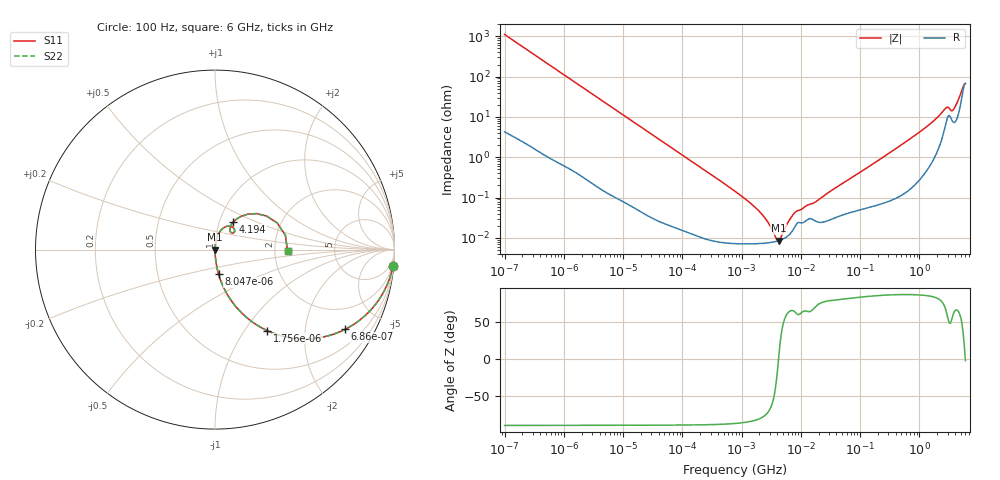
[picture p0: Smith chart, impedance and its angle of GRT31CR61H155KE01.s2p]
!Murata Part Number: GRT31CR61H155KE01
!These Parameters are Measured in Series Mode Connection
!Data Generated on Jun 19, 2026
!  o--ll--o
!Port1  Port2
!  o------o
!Operation Temp=25[degC], DC Bias Voltage=0[V]
!Freq. Start=100[Hz] Stop=6[GHz] 401[Steps]
# Hz S RI R 50
!Freq.(Hz) S11(Real) S11(Imag) S21(Real) S21(Imag) S12(Real) S12(Imag) S22(Real) S22(Imag)
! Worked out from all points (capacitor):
!   401 points, 100 Hz to 6 GHz, reference 50 ohm
!   read as one part in series: C = 1.43 uF near 109 Hz
!   lowest |Z| = 8.57 mohm at 4.246 MHz (marker M1)
!   series resonance near 4.206 MHz, so ESL is about 1 nH
!   S11 on the Smith chart (normalised r, x): 100 Hz: 1, -22; 686 Hz: 1.02, -3.26; 1.756 kHz: 1.01, -1.28; 8.047 kHz: 1.00, -0.28; 4.194 GHz: 1.16, +0.37; 6 GHz: 2.36, -0.05
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100  0.9916 -0.0891  0.00835 0.0891  0.00835 0.0891  0.9916 -0.0891
320  0.9229 -0.2645  0.0771 0.2645  0.0771 0.2645  0.9229 -0.2645
686  0.7258 -0.4436  0.2742 0.4436  0.2742 0.4436  0.7258 -0.4436
1756  0.2912 -0.4514  0.7088 0.4514  0.7088 0.4514  0.2912 -0.4514
2008  0.2395 -0.4238  0.7605 0.4238  0.7605 0.4238  0.2395 -0.4238
3594  0.0907 -0.2842  0.9093 0.2842  0.9093 0.2842  0.0907 -0.2842
8047  0.0202 -0.1373  0.9798 0.1373  0.9798 0.1373  0.0202 -0.1373
40335  0.00105 -0.0281  0.999 0.0281  0.999 0.0281  0.00105 -0.0281
774597  7.41e-05 -0.00143  0.9999 0.00143  0.9999 0.00143  7.41e-05 -0.00143
1983483  7.25e-05 -0.000452  0.9999 0.000452  0.9999 0.000452  7.25e-05 -0.000452
2713602  7.51e-05 -0.000249  0.9999 0.000249  0.9999 0.000249  7.51e-05 -0.000249
3712478  8.11e-05 -6.94e-05  0.9999 6.94e-05  0.9999 6.94e-05  8.11e-05 -6.94e-05
4246196  8.55e-05 5.4e-06  0.9999 -5.4e-06  0.9999 -5.4e-06  8.55e-05 5.4e-06
7947587  0.000191 0.000381  0.9998 -0.000381  0.9998 -0.000381  0.000191 0.000381
1.555665e7  0.000292 0.000647  0.9997 -0.000647  0.9997 -0.000647  0.000292 0.000647
3.124326e8  0.000978 0.0127  0.999 -0.0127  0.999 -0.0127  0.000978 0.0127
1.309207e9  0.00756 0.0556  0.9924 -0.0556  0.9924 -0.0556  0.00756 0.0556
2.679998e9  0.067 0.1299  0.933 -0.1299  0.933 -0.1299  0.067 0.1299
3.666503e9  0.0833 0.1052  0.9167 -0.1052  0.9167 -0.1052  0.0833 0.1052
4.193612e9  0.1023 0.1542  0.8977 -0.1542  0.8977 -0.1542  0.1023 0.1542
5.016141e9  0.2303 0.2005  0.7697 -0.2005  0.7697 -0.2005  0.2303 0.2005
6e9  0.4044 -0.00921  0.5956 0.00921  0.5956 0.00921  0.4044 -0.00921
